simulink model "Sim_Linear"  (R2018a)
settings: Solver=ode3  StartTime=0.0  StopTime=30000  FixedStep=Ts  RelTol=1e-3  EnableMultiTasking=on
InitFcn:
  | run
StopFcn:
  | pl
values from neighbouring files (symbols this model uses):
  atto = [0, 0, -0]'*d2r    [run.m]
  ini = [wb0; atto; Hco]    [run.m]
  Kq1 = I22*ww^2 - 3*wo2*(I11-I33)    [run.m]
  Kq2 = 2*I22*zet*ww    [run.m]
  Kqi = 0.0005    [run.m]
  Kr1 = (0.1*I11*I33*zet^2/Hy0) - sqrt( ((0.01^zet^4*I11^2*I33^2)/Hy0^2)+(4*I11*I33*zet^2) )    [run.m]
  Kr2 = 0.05*Kr1    [run.m]
  Kr3 = 0.04*zet*(Kr2-Hy0) * sqrt(abs(Hy0/(I11*I33)))    [run.m]
  Tbs = (wo2)*[-2*I32, 3*I31, -I12]'    [run.m]
  Ts = 0.001    [run.m]    (also in runf.m = 0.0005)
  wb0 = [0.0, -wo, 0.0]'    [run.m]
undefined symbols (not defined in the file or in its folder): den, DiscIntNeverNeededParam, num, Spacecraft, Wheel_Dynamics
libraries: simulink x3

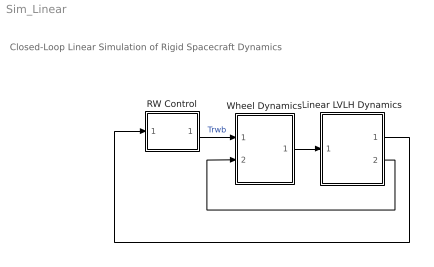
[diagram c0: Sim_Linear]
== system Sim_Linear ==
  note: Closed-Loop Linear Simulation of Rigid Spacecraft Dynamics
  Linear LVLH Dynamics : Subsystem
  RW Control : Subsystem
  Wheel Dynamics : Subsystem
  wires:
  RW Control/1(Tc) -> Wheel Dynamics/1(Twi)  "Trwb"
  Wheel Dynamics/1(Tcb) -> Linear LVLH Dynamics/1(Tsc)
  Linear LVLH Dynamics/2(wb) -> Wheel Dynamics/2(wb)
  Linear LVLH Dynamics/1(attit) -> RW Control/1(atti)

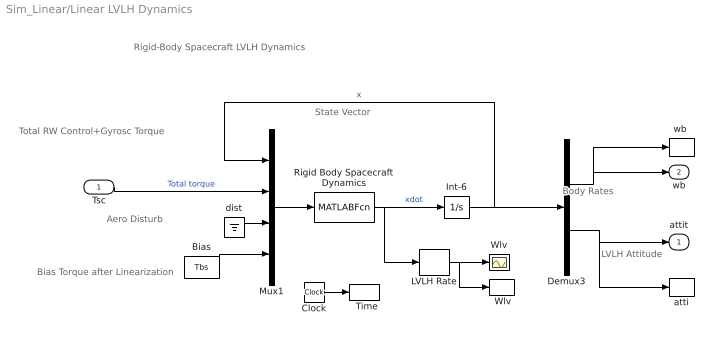
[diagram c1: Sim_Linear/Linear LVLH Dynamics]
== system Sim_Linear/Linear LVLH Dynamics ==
  note: LVLH Attitude
  note: Body Rates
  note: Bias Torque after Linearization
  note: Aero Disturb
  note: Total RW Control+Gyrosc Torque
  note: State Vector
  note: Rigid-Body Spacecraft LVLH Dynamics
  Tsc : Inport
  "  Time" : ToWorkspace  VariableName=time  SampleTime=-1
  "  Wlv " : ToWorkspace  VariableName=Wlv  SampleTime=-1
  Bias : Constant  Value=Tbs
  Clock : Clock
  Demux3 : Demux  Outputs=[3, 3]
  Int-6 : Integrator  InitialCondition=ini
  LVLH Rate : Selector  InputPortWidth=6  IndexOptions=Index vector (dialog)  Indices=[4:6]  OutputSizes=1
  Mux1 : Mux  Inputs=[6, 3, 3, 3]
  Rigid Body Spacecraft Dynamics : MATLABFcn  MATLABFcn=Spacecraft( u(1:6), u(7:9) , u(10:12), u(13:15) )  OutputDimensions=6
  Wlv : Scope
  atti : ToWorkspace  VariableName=atti  SampleTime=-1
  dist : Ground
  "wb " : ToWorkspace  VariableName=wb  SampleTime=-1
  attit : Outport
  wb : Outport  Port=2
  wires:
  dist/1 -> Mux1/3
  Bias/1 -> Mux1/4
  LVLH Rate/1 -> Wlv/1, "  Wlv "/1
  Rigid Body Spacecraft Dynamics/1 -> LVLH Rate/1, Int-6/1  "xdot"
  Tsc/1 -> Mux1/2  "Total torque"
  Int-6/1 -> Demux3/1, Mux1/1  "x"
  Demux3/1 -> "wb "/1, wb/1
  Demux3/2 -> atti/1, attit/1
  Mux1/1 -> Rigid Body Spacecraft Dynamics/1
  Clock/1 -> "  Time"/1

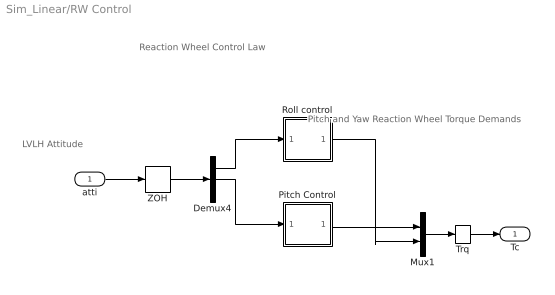
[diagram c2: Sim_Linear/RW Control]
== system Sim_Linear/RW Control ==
  note: Pitch and Yaw Reaction Wheel Torque Demands
  note: LVLH Attitude
  note: Reaction Wheel Control Law
  atti : Inport
  Demux4 : Demux  Outputs=3
  Mux1 : Mux  Inputs=2
  Pitch Control : Subsystem
  Roll control : Subsystem
  Trq : Memory
  ZOH : ZeroOrderHold  SampleTime=Ts
  Tc : Outport
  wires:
  Demux4/1 -> Roll control/1(phi)
  Pitch Control/1(Tcy) -> Mux1/1
  Demux4/2 -> Pitch Control/1(the)
  atti/1 -> ZOH/1
  Mux1/1 -> Trq/1
  Roll control/1(Tcz) -> Mux1/2
  Trq/1 -> Tc/1
  ZOH/1 -> Demux4/1

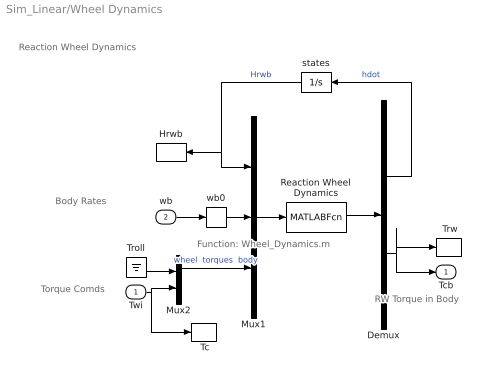
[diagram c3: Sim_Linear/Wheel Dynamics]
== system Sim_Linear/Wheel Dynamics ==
  note: Torque Comds
  note: RW Torque in Body
  note: Body Rates
  note: Reaction Wheel Dynamics
  note: Function: Wheel_Dynamics.m
  Twi : Inport
  wb : Inport  Port=2
  " Tc" : ToWorkspace  VariableName=Tc  SampleTime=-1
  " Trw" : ToWorkspace  VariableName=Trw  SampleTime=-1
  Demux : Demux  Outputs=[3, 3]
  Hrwb : ToWorkspace  VariableName=Hrwb  SampleTime=-1
  Mux1 : Mux  Inputs=[3, 3, 3]
  Mux2 : Mux  Inputs=[1,2]
  Reaction Wheel Dynamics : MATLABFcn  MATLABFcn=Wheel_Dynamics( u(1:3), u(4:6), u(7:9) )  OutputDimensions=3+3
  Troll : Ground
  states : Integrator
  wb0 : Memory  InitialCondition=wb0
  Tcb : Outport
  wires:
  wb0/1 -> Mux1/2
  Troll/1 -> Mux2/1
  Twi/1 -> Mux2/2, " Tc"/1
  Mux1/1 -> Reaction Wheel Dynamics/1
  Reaction Wheel Dynamics/1 -> Demux/1
  Demux/2 -> Tcb/1, " Trw"/1
  Mux2/1 -> Mux1/3  "wheel  torques  body"
  wb/1 -> wb0/1
  Demux/1 -> states/1  "hdot"
  states/1 -> Mux1/1, Hrwb/1  "Hrwb"

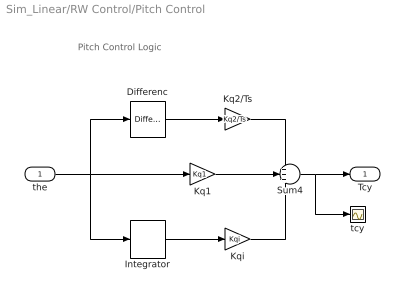
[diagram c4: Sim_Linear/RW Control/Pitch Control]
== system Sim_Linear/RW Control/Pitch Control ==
  note: Pitch Control Logic
  the : Inport
  Differenc : simulink/Discrete/Difference  ICPrevInput=atto(2)  InputProcessing=Inherited  OutMin=[]  OutMax=[]  OutDataType=sfix(16)  OutScaling=2^-10  DoSatur=off
  Integrator : DiscreteIntegrator  InitialCondition=atto(2)  SampleTime=Ts  ICPrevOutput=DiscIntNeverNeededParam  ICPrevScaledInput=DiscIntNeverNeededParam
  Kq1 : Gain  Gain=Kq1
  Kq2/Ts : Gain  Gain=Kq2/Ts
  Kqi : Gain  Gain=Kqi
  Sum4 : Sum  Inputs=+++
  tcy : Scope
  Tcy : Outport
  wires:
  Kq1/1 -> Sum4/2
  Sum4/1 -> Tcy/1, tcy/1
  Kq2/Ts/1 -> Sum4/1
  the/1 -> Kq1/1, Integrator/1, Differenc/1
  Kqi/1 -> Sum4/3
  Integrator/1 -> Kqi/1
  Differenc/1 -> Kq2/Ts/1

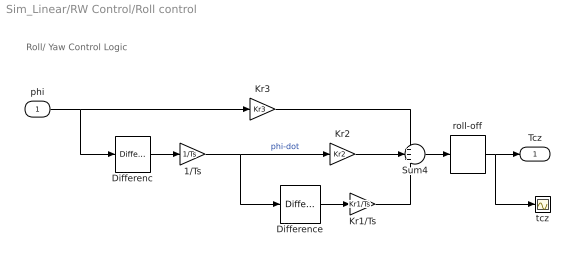
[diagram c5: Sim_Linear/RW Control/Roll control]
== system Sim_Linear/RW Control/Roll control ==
  note: Roll/ Yaw Control Logic
  phi : Inport
  1/Ts : Gain  Gain=1/Ts
  Differenc : simulink/Discrete/Difference  ICPrevInput=atto(1)  InputProcessing=Inherited  OutMin=[]  OutMax=[]  OutDataType=sfix(16)  OutScaling=2^-10  DoSatur=off
  Difference : simulink/Discrete/Difference  ICPrevInput=0.0  InputProcessing=Inherited  OutMin=[]  OutMax=[]  OutDataType=sfix(16)  OutScaling=2^-10  DoSatur=off
  Kr1/Ts : Gain  Gain=Kr1/Ts
  Kr2 : Gain  Gain=Kr2
  Kr3 : Gain  Gain=Kr3
  Sum4 : Sum  Inputs=+++
  roll-off : DiscreteTransferFcn  Numerator=[num]  Denominator=[den]  SampleTime=Ts
  tcz : Scope
  Tcz : Outport
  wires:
  Kr3/1 -> Sum4/1
  Kr2/1 -> Sum4/2
  Kr1/Ts/1 -> Sum4/3
  phi/1 -> Kr3/1, Differenc/1
  Sum4/1 -> roll-off/1
  Difference/1 -> Kr1/Ts/1
  Differenc/1 -> 1/Ts/1
  1/Ts/1 -> Kr2/1, Difference/1  "phi-dot"
  roll-off/1 -> Tcz/1, tcz/1
